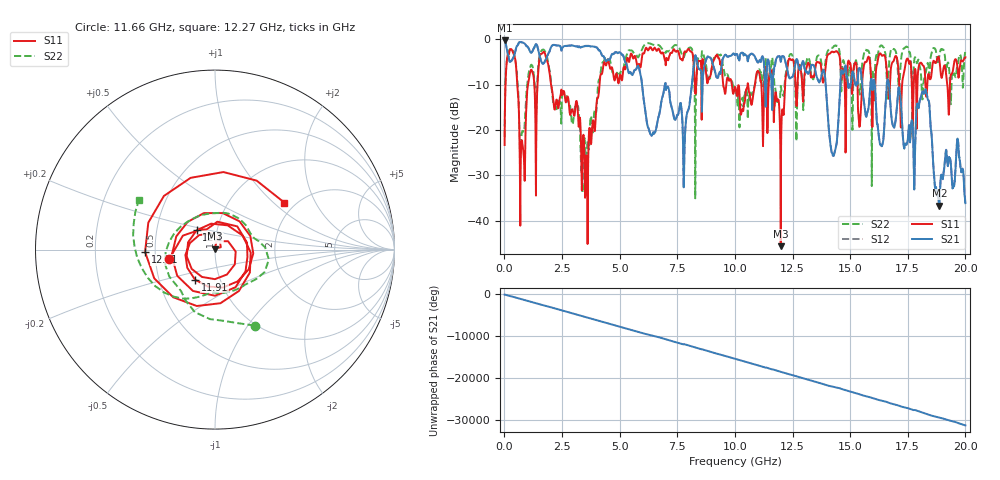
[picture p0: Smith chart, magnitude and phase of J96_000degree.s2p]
!Keysight Technologies,N5222A,MY51421036,A.10.65.16
!Date: Friday, March 31, 2023 14:22:12
!Correction: S11(Full 2 Port(1,2))
!S21(Full 2 Port(1,2))
!S12(Full 2 Port(1,2))
!S22(Full 2 Port(1,2))
!S2P File: Measurements: S11, S21, S12, S22:
# Hz S  dB  R 50
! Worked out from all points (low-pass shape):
!   2000 points, 10 MHz to 20 GHz, reference 50 ohm
!   highest |S21| = -0.25 dB at 10 MHz (marker M1); lowest = -36.7 dB at 18.87 GHz (marker M2)
!   |S21| within 3 dB of the highest: 438.3 MHz to 1.509 GHz (1.071 GHz wide, 110 % of centre); 1.898 GHz to 4.209 GHz (2.311 GHz wide, 75.7 % of centre)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
!   lowest |S11| = -45.6 dB at 11.99 GHz (marker M3), VSWR 1.01, Z = 49.9 + j0.516 ohm
!   |S11| at or under -10 dB: 2.025 GHz to 4.123 GHz (2.098 GHz wide, 68.2 % of centre); 9.868 GHz to 10.55 GHz (684.1 MHz wide, 6.7 % of centre); 11.65 GHz to 12.18 GHz (524.7 MHz wide, 4.4 % of centre)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
!   |S22| runs from -35.1 to -0.8 dB; largest |S21 - S12| = 0.011
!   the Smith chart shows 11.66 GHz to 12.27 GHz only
!   S11 on the Smith chart (normalised r, x): 11.66 GHz: 0.59, -0.07; 11.91 GHz: 0.76, -0.26; 12.1 GHz: 0.80, +0.18; 12.21 GHz: 0.44, -0.01; 12.27 GHz: 1.75, +1.18
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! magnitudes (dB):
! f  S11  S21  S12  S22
! 10 MHz  -23.3  -0.2  -0.3  -21.6
! 380 MHz  -3.0  -4.1  -4.1  -2.6
! 780 MHz  -23.1  -0.7  -0.7  -20.2
! 1.71 GHz  -2.8  -5.3  -5.3  -2.3
! 3.35 GHz  -30.9  -1.7  -1.6  -29.7
! 4.33 GHz  -5.1  -4.0  -3.9  -4.7
! 6.68 GHz  -2.1  -17.3  -17.2  -1.3
! 10.01 GHz  -10.5  -3.4  -3.5  -10.7
! 11.66 GHz  -11.7  -8.2  -8.2  -6.4
! 11.91 GHz  -13.9  -3.7  -3.7  -13.2
! 11.99 GHz  -45.6  -5.0  -5.0  -10.3
! 12.1 GHz  -16.6  -3.7  -3.8  -12.5
! 12.21 GHz  -8.2  -5.3  -5.3  -7.5
! 12.27 GHz  -6.6  -6.6  -6.6  -5.9
! 13.34 GHz  -8.2  -5.6  -5.6  -8.2
! 14.26 GHz  -2.8  -25.7  -25.6  -1.7
! 14.71 GHz  -6.7  -7.5  -7.5  -4.6
! 16.34 GHz  -3.3  -23.4  -23.4  -1.3
! 16.67 GHz  -12.0  -9.4  -9.4  -7.2
! 18.32 GHz  -12.3  -12.0  -11.9  -6.2
! 18.87 GHz  -4.6  -36.7  -36.2  -3.6
! 20 GHz  -4.0  -36.1  -36.2  -2.6
